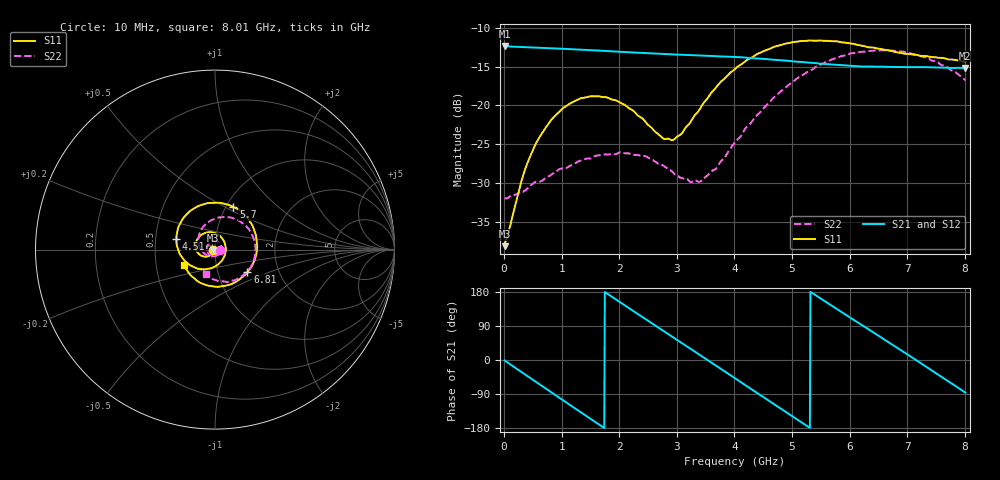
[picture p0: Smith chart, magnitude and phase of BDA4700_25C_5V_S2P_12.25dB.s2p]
!Agilent Technologies,E5071B,MY42404982,A.09.10
!Date: Mon Oct 20 13:32:15 2025
!Data & Calibration Information:
!Freq	S11:SOLT2(ON)	S21:SOLT2(ON)	S12:SOLT2(ON)	S22:SOLT2(ON)
# Hz S RI R 50
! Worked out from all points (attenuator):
!   801 points, 10 MHz to 8.01 GHz, reference 50 ohm
!   highest |S21| = -12.35 dB at 10 MHz (marker M1); lowest = -15.2 dB at 8 GHz (marker M2)
!   lowest |S11| = -38.1 dB at 10 MHz (marker M3), VSWR 1.03, Z = 48.8 - j0.166 ohm
!   |S11| at or under -10 dB: start of sweep to end of sweep
!   |S22| runs from -32.0 to -12.9 dB; largest |S21 - S12| = 0.0017
!   S11 on the Smith chart (normalised r, x): 10 MHz: 0.98, -0.00; 4.51 GHz: 0.64, +0.08; 5.7 GHz: 1.08, +0.55; 6.81 GHz: 1.39, -0.36; 8.01 GHz: 0.70, -0.12
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1e7  -0.0123 -0.0017  0.2411 -0.0053  0.241 -0.00556  0.0252 -0.00101
3.4e8  -0.0239 -0.0272  0.1926 -0.1387  0.1926 -0.1389  0.0219 -0.0175
5.6e8  -0.0427 -0.0384  0.1231 -0.2009  0.1229 -0.201  0.0139 -0.029
8.8e8  -0.0787 -0.0331  -0.00609 -0.2326  -0.00623 -0.2328  -0.00986 -0.0356
1.35e9  -0.1093 0.0217  -0.1743 -0.1475  -0.1743 -0.1476  -0.042 -0.0139
1.65e9  -0.0934 0.0659  -0.2222 -0.0376  -0.2222 -0.0376  -0.0458 0.0132
1.94e9  -0.0536 0.0935  -0.2091 0.0757  -0.2091 0.0758  -0.0317 0.0367
2.33e9  0.0137 0.0845  -0.1112 0.1877  -0.1114 0.1877  0.00137 0.0478
2.68e9  0.0547 0.0353  0.0169 0.2146  0.0168 0.2145  0.028 0.0314
2.95e9  0.0571 -0.0193  0.1117 0.1813  0.1116 0.181  0.0351 0.00953
3.4e9  -0.00311 -0.0945  0.2041 0.0481  0.2043 0.048  0.0166 -0.0276
4.01e9  -0.1537 -0.0758  0.1364 -0.153  0.1365 -0.1529  -0.0492 -0.0298
4.51e9  -0.2153 0.061  -0.0309 -0.1969  -0.0307 -0.1972  -0.0907 0.0323
4.97e9  -0.152 0.2024  -0.1584 -0.1102  -0.1585 -0.1107  -0.0727 0.1173
5.35e9  -0.0284 0.2599  -0.1876 0.0103  -0.1877 0.00972  -0.00417 0.17
5.7e9  0.1022 0.2376  -0.145 0.1121  -0.145 0.1124  0.0854 0.1791
6.21e9  0.2246 0.0917  -0.00809 0.1776  -0.00641 0.178  0.1987 0.0973
6.68e9  0.2101 -0.0839  0.1221 0.1279  0.1225 0.1279  0.2225 -0.0327
6.81e9  0.1809 -0.1249  0.147 0.0976  0.1476 0.0969  0.2125 -0.0682
7.36e9  0.00248 -0.2068  0.1645 -0.0629  0.1646 -0.063  0.1067 -0.1725
8e9  -0.171 -0.0884  0.0146 -0.1735  0.0148 -0.1739  -0.0505 -0.1374
8.01e9  -0.1723 -0.0857  0.0114 -0.1738  0.0119 -0.1739  -0.0526 -0.1351
